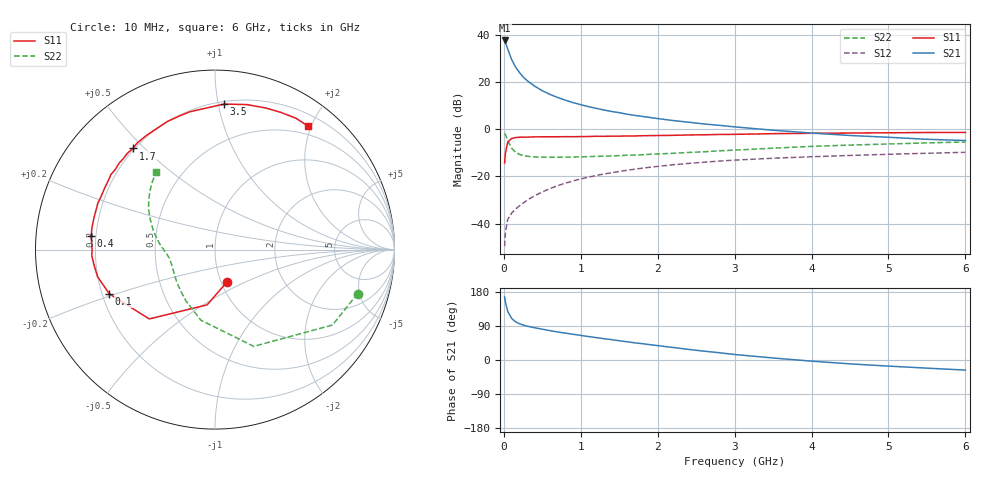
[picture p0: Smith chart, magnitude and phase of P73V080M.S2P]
! SIEMENS Small Signal Semiconductors
! BFP196
! Si NPN RF Bipolar Junction Transistor in SOT143
! VCE = 3 V  IC = 80 mA
! Common Emitter S-Parameters:  May  1996
# GHz  S  MA  R  50
!  f  S11  S21  S12  S22
! GHz  MAG  ANG  MAG  ANG  MAG  ANG  MAG  ANG
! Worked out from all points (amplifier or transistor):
!   36 points, 10 MHz to 6 GHz, reference 50 ohm
!   highest |S21| = 37.8 dB at 10 MHz (marker M1)
!   |S21| within 3 dB of that: start of sweep to 43.71 MHz
!   unconditionally stable (mu >= 1): 345.2 MHz to 4.744 GHz
!   at 250 MHz: K = 0.93, MSG = 26.9 dB, |S12| = -31.3 dB
!   at 1.4 GHz: K = 1.09, MAG = 11.2 dB, |S12| = -18.4 dB
!   at 6 GHz: K = 0.98, MSG = 2.5 dB, |S12| = -9.7 dB
!   S11 on the Smith chart (normalised r, x): 10 MHz: 1.06, -0.40; 100 MHz: 0.23, -0.19; 400 MHz: 0.18, +0.05; 1.7 GHz: 0.19, +0.46; 3.5 GHz: 0.22, +1.04; 6 GHz: 0.37, +1.96
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0.01  0.1938 -70.5  77.76 166.6  0.0033 75.8  0.832 -17.1
0.02  0.3109 -98.1  71.29 153.7  0.0064 68.0  0.7777 -32.7
0.05  0.5324 -133.5  51.4 128.8  0.0122 55.4  0.5808 -68.2
0.1  0.6383 -157.3  30.84 110.0  0.0165 51.2  0.4011 -101.3
0.15  0.6716 -167.0  21.5 101.2  0.0201 54.1  0.3284 -119.5
0.2  0.6797 -172.9  16.4 96.0  0.0235 57.6  0.2961 -131.2
0.25  0.6871 -177.1  13.12 92.3  0.0271 59.9  0.2787 -139.8
0.3  0.6848 179.5  10.99 89.5  0.0311 62.4  0.2692 -145.5
0.4  0.6939 173.8  8.317 85.1  0.0389 64.8  0.2598 -153.7
0.5  0.6967 169.7  6.649 81.3  0.0468 65.6  0.2563 -158.9
0.6  0.697 165.4  5.547 77.5  0.0554 66.0  0.2557 -162.5
0.7  0.6988 161.4  4.774 73.9  0.0636 65.9  0.2564 -165.1
0.9  0.7005 154.6  3.712 67.9  0.0806 64.1  0.2585 -169.4
1.1  0.7067 147.9  3.051 61.9  0.0965 61.9  0.2645 -172.2
1.4  0.7191 138.0  2.405 53.7  0.1197 57.8  0.2731 -176.1
1.7  0.726 129.1  1.989 45.3  0.1427 53.4  0.2857 179.9
2.2  0.7485 115.6  1.545 33.0  0.177 45.7  0.3106 173.8
3  0.7853 96.1  1.132 14.5  0.2226 33.5  0.3631 162.0
3.5  0.8123 86.4  0.961 5.3  0.2441 26.4  0.3993 154.8
4.5  0.8377 70.5  0.743 -10.2  0.28 14.3  0.4645 142.5
5.5  0.8598 58.3  0.617 -21.5  0.3117 3.5  0.5168 132.3
6  0.8616 52.8  0.581 -26.6  0.3263 -2.3  0.5412 127.3
